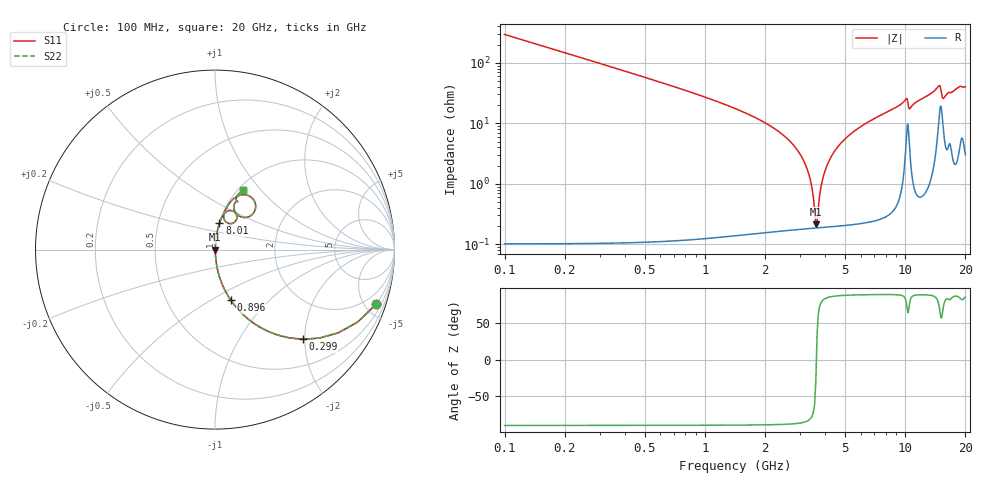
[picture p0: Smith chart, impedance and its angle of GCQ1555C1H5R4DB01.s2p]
!Murata Part Number: GCQ1555C1H5R4DB01
!These Parameters are Measured in Series Mode Connection
!Data Generated on Mar 13, 2026
!  o--ll--o
!Port1  Port2
!  o------o
!Operation Temp=25[degC], DC Bias Voltage=0[V]
!Freq. Start=100[MHz] Stop=20[GHz] 401[Steps]
# Hz S RI R 50
!Freq.(Hz) S11(Real) S11(Imag) S21(Real) S21(Imag) S12(Real) S12(Imag) S22(Real) S22(Imag)
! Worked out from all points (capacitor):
!   401 points, 100 MHz to 20 GHz, reference 50 ohm
!   read as one part in series: C = 5.4 pF near 199.5 MHz
!   lowest |Z| = 214 mohm at 3.583 GHz (marker M1)
!   series resonance near 3.606 GHz, so ESL is about 360 pH
!   S11 on the Smith chart (normalised r, x): 100 MHz: 1.00, -5.89; 299 MHz: 1.00, -1.96; 896 MHz: 1.00, -0.62; 8.01 GHz: 1.01, +0.30; 20 GHz: 1.06, +0.81
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1e8  0.8965 -0.3044  0.1035 0.3044  0.1035 0.3044  0.8965 -0.3044
2.99e8  0.4893 -0.4994  0.5107 0.4994  0.5107 0.4994  0.4893 -0.4994
5.4775e8  0.2169 -0.4111  0.7831 0.4111  0.7831 0.4111  0.2169 -0.4111
8.96e8  0.0878 -0.281  0.9122 0.281  0.9122 0.281  0.0878 -0.281
2.7865e9  0.00353 -0.0424  0.9965 0.0424  0.9965 0.0424  0.00353 -0.0424
3.1845e9  0.00221 -0.0203  0.9978 0.0203  0.9978 0.0203  0.00221 -0.0203
3.43325e9  0.0019 -0.008  0.9981 0.008  0.9981 0.008  0.0019 -0.008
3.5825e9  0.00186 -0.00106  0.9981 0.00106  0.9981 0.00106  0.00186 -0.00106
3.682e9  0.00188 0.00341  0.9981 -0.00341  0.9981 -0.00341  0.00188 0.00341
3.83125e9  0.00199 0.0099  0.998 -0.0099  0.998 -0.0099  0.00199 0.0099
3.9805e9  0.00217 0.0162  0.9978 -0.0162  0.9978 -0.0162  0.00217 0.0162
4.42825e9  0.00311 0.0338  0.9969 -0.0338  0.9969 -0.0338  0.00311 0.0338
5.32375e9  0.00639 0.0654  0.9936 -0.0654  0.9936 -0.0654  0.00639 0.0654
6.7665e9  0.0147 0.1102  0.9853 -0.1102  0.9853 -0.1102  0.0147 0.1102
8.01025e9  0.0248 0.1463  0.9752 -0.1463  0.9752 -0.1463  0.0248 0.1463
1.005e10  0.0843 0.2176  0.9157 -0.2176  0.9157 -0.2176  0.0843 0.2176
1.05475e10  0.0601 0.1553  0.9399 -0.1553  0.9399 -0.1553  0.0601 0.1553
1.338325e10  0.0948 0.2752  0.9052 -0.2752  0.9052 -0.2752  0.0948 0.2752
1.49255e10  0.2263 0.2493  0.7737 -0.2493  0.7737 -0.2493  0.2263 0.2493
1.5423e10  0.1322 0.1884  0.8678 -0.1884  0.8678 -0.1884  0.1322 0.1884
1.67165e10  0.1263 0.2677  0.8737 -0.2677  0.8737 -0.2677  0.1263 0.2677
2e10  0.1583 0.3294  0.8417 -0.3294  0.8417 -0.3294  0.1583 0.3294
